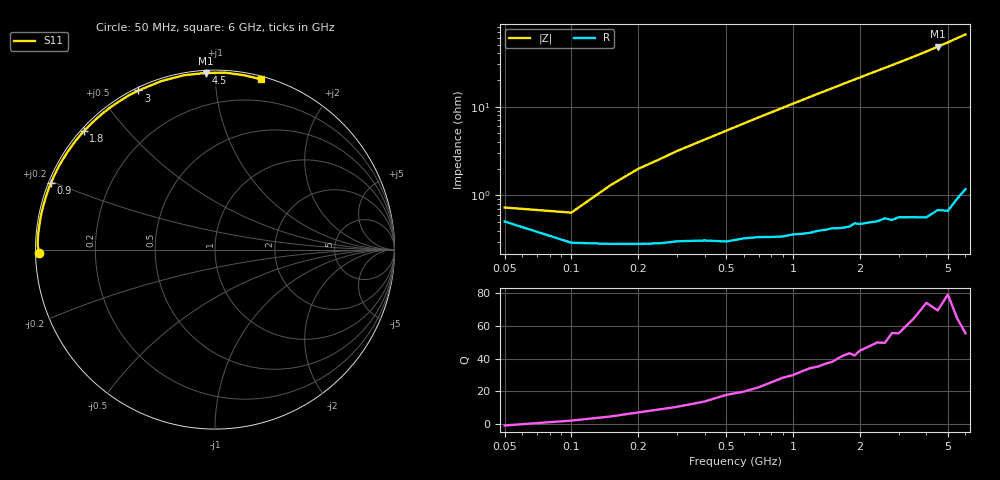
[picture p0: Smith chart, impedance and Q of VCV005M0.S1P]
! Infineon Technologies  Discrete & RF Semiconductors
! BBY 56-03
! Si Tuning Diode in SOD323
! VR =
! S-Parameters:  June  1999
# GHz  S  MA  R  50
!  f  S11
! GHz  MAG  ANG
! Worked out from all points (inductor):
!   34 points, 50 MHz to 6 GHz, reference 50 ohm
!   read as one part to ground: L = 1.56 nH near 150 MHz
!   highest Q = 74.2 at 4.5 GHz (marker M1), where L = 1.68 nH
!   S11 on the Smith chart (normalised r, x): 50 MHz: 0.01, -0.01; 900 MHz: 0.01, +0.19; 1.8 GHz: 0.01, +0.38; 3 GHz: 0.01, +0.63; 4.5 GHz: 0.01, +0.95; 6 GHz: 0.02, +1.30
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0.05  0.9799 -178.8
0.1  0.9884 178.7
0.2  0.9888 175.5
0.3  0.988 172.8
0.5  0.9881 167.8
0.7  0.9869 162.8
0.8  0.9869 160.4
0.9  0.9868 158.0
1  0.9863 155.6
1.1  0.9862 153.3
1.2  0.9859 151.0
1.3  0.9853 148.7
1.5  0.9847 144.3
1.6  0.9849 142.2
1.7  0.9848 140.0
1.8  0.9846 137.9
2  0.984 133.9
2.2  0.9839 129.9
2.4  0.9839 126.2
2.6  0.9832 122.6
2.8  0.9844 119.1
3  0.9839 115.7
3.5  0.9853 107.7
4  0.9868 100.1
4.5  0.9858 93.0
5  0.9875 86.6
5.5  0.9849 80.4
6  0.9828 75.0
